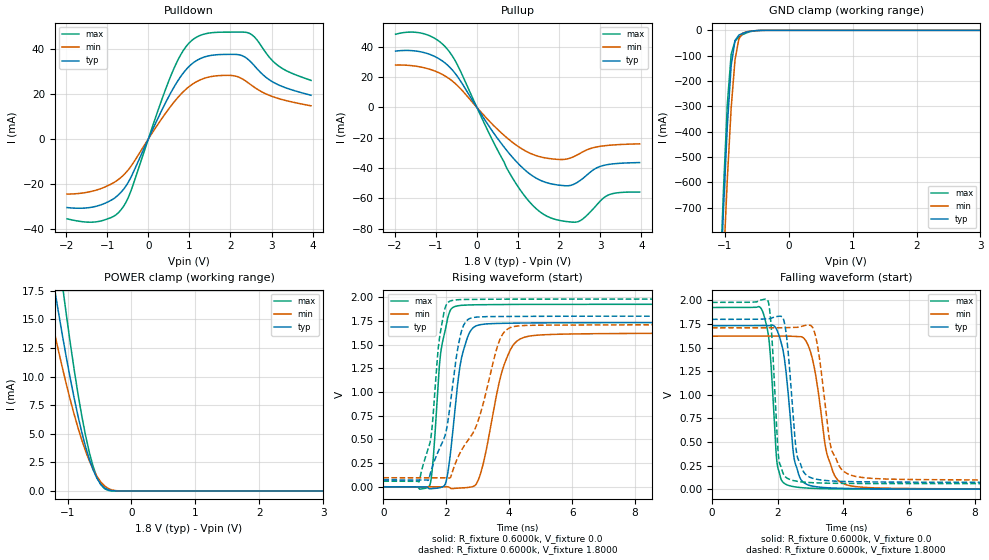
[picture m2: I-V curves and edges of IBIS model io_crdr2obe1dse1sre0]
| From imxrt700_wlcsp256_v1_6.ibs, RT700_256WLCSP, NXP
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[Model] io_crdr2obe1dse1sre0
|   Model io_crdr2obe1dse1sre0
| This model was characterised for following simulation conditions:
| External (pad) voltage:
|   - Typ: 1.8V,   - Min: 1.71V,   - Max: 1.98V
| Library cells for typ/min/max conditions are connected as defined below:
|  PAD_IO - External Pad
|  ipp_do - Core Input
|  ipp_obe - Output Buffer Enable
|  ASRCN3V3[3] - NC
|  ASRCN3V3[4] - NC
|  ASRCP3V3[4] - NC
|  REFAPBIAS3V3 - gnde
|  REFBAMPL3V3 - vdd1v8
|  REFCAMPH3V3 - vdd1v8
|  REFDNBIAS3V3 - vdd1v8
|  REFH3V3 - REFH3V3
|  REFL3V3 - REFL3V3
|  gnde - gnde
|  ipp_dse - vdd
|  ipp_ina235_3v - NC
|  ipp_ina40_3v - NC
|  ipp_ina_mux - NC
|  ipp_ind - NC
|  ipp_ind_1p8v - NC
|  ipp_ind_3v - NC
|  ipp_sre - gnde
|  vdd - vdd
|  vdd1v8 - vdd1v8
|  vdda - vdde3v3
|  vdde3v3 - vdde3v3
| All other pins connected to ground
Model_type I/O
Polarity   Non-Inverting
Enable   Active-High
Vinl =   0.5400V
Vinh =   1.2600V
Vmeas =  0.9000V
Cref =   15.0000pF
Rref =   0.6000k
Vref =   0.0V
C_comp   3.9792pF   3.7942pF   4.1043pF
|C_comp_pullup   0.4868pF   0.5823pF   0.4754pF
|C_comp_pulldown   2.0823pF   2.1675pF   1.8519pF
[Model Spec]
| variable   typ   min   max
Vinh   1.2600V   NA   NA
Vinl   0.5400V   NA   NA
Vref   0.0V   0.0V   0.0V
Cref   15.0000pF   15.0000pF   15.0000pF
Rref   0.6000k   0.6000k   0.6000k
[Receiver Thresholds]
Vcross_high  =   0.0V
Vcross_low  =   0.0V
Vdiff_ac  =   0.0V
Vdiff_dc  =   0.0V
Tdiffslew_ac  =   0.0S
[Temperature Range]   25.0000   0.1250k   -40.0000
[Voltage Range]   1.8000V   1.7100V   1.9800V
[Pullup Reference]   1.8000V   1.7100V   1.9800V
[Pulldown Reference]   0.0V   0.0V   0.0V
[POWER Clamp Reference]   1.8000V   1.7100V   1.9800V
[GND Clamp Reference]   0.0V   0.0V   0.0V
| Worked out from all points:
|   slope of the pulldown table from 0 to 0.27 V, typ, clamps not added: 25.6 ohm
|   slope of the pullup table from 0 to 0.27 V, typ, clamps not added: 23.8 ohm
|   GND clamp passes 1 mA (typ) near -0.50 V on its own axis
|   POWER clamp passes 1 mA (typ) near -0.53 V on its own axis
|   rising waveform, R_fixture 0.6000k, V_fixture 0.0: 20-80 % time 373ps typ, 622ps min, 283ps max; typ from 0 V to 1.73 V
|   rising waveform, R_fixture 0.6000k, V_fixture 1.8000: 20-80 % time 558ps typ, 1ns min, 331ps max; typ from 0.072 V to 1.8 V
|   falling waveform, R_fixture 0.6000k, V_fixture 0.0: 20-80 % time 288ps typ, 434ps min, 205ps max; typ from 1.73 V to 0 V
|   falling waveform, R_fixture 0.6000k, V_fixture 1.8000: 20-80 % time 243ps typ, 371ps min, 176ps max; typ from 1.8 V to 0.072 V
[Pulldown]
|Voltage   I(typ)   I(min)   I(max)
-1.98V    -30.4mA    -24.44mA   -35.4mA
-1.2V     -29.48mA   -22.28mA   -36.54mA
-840mV    -26.45mA   -19.34mA   -34.25mA
-600mV    -22.26mA   -15.94mA   -29.79mA
-420mV    -16.87mA   -12.03mA   -22.87mA
600mV     22.22mA    15.79mA    30.28mA
900mV     30.36mA    21.79mA    40.52mA
1.14V     34.38mA    25.06mA    44.79mA
1.98V     37.51mA    28.2mA     47.38mA
2.46V     34.79mA    24.52mA    46.85mA
3.12V     24.4mA     18.2mA     33.06mA
3.96V     19.37mA    14.7mA     25.97mA
[Pullup]
|Voltage   I(typ)   I(min)   I(max)
-1.98V    37.17mA    27.99mA    48.3mA
-1.26V    36mA       26.04mA    48.37mA
-720mV    28.06mA    19.81mA    38.46mA
-480mV    20.65mA    14.61mA    28.37mA
780mV     -30.13mA   -21.13mA   -42.58mA
1.2V      -41.94mA   -28.92mA   -59.68mA
1.62V     -48.87mA   -33.02mA   -70.4mA
2.16V     -51.62mA   -34.11mA   -75.13mA
2.46V     -49.1mA    -31.02mA   -75.32mA
2.88V     -40.32mA   -26.22mA   -65.36mA
3.18V     -37.66mA   -25.01mA   -57.94mA
3.96V     -36.33mA   -23.97mA   -55.79mA
[GND_clamp]
|Voltage   I(typ)   I(min)   I(max)
-1.98V    -7.543A    -7.6A      -7.897A
-1.08V    -1.077A    -1.286A    -1.025A
-1.02V    -705.3mA   -921.3mA   -628.8mA
-960mV    -377.1mA   -587.4mA   -291.7mA
-900mV    -139.2mA   -307mA     -94.38mA
-840mV    -40.12mA   -117mA     -42.82mA
-780mV    -18.81mA   -33.95mA   -26.13mA
-720mV    -11.86mA   -11.44mA   -16.78mA
-660mV    -7.061mA   -5.737mA   -9.992mA
-540mV    -1.684mA   -1.901mA   -2.15mA
-420mV    -207.1uA   -403.7uA   -160.6uA
3.96V     0A         0A         0A
[POWER_clamp]
|Voltage   I(typ)   I(min)   I(max)
-1.98V    46.79mA    35.94mA    61.38mA
-1.32V    21.77mA    16.85mA    28.91mA
-1.2V     17.57mA    13.71mA    23.33mA
-1.14V    15.55mA    12.2mA     20.62mA
-1.08V    13.59mA    10.75mA    17.99mA
-1.02V    11.7mA     9.353mA    15.46mA
-900mV    8.209mA    6.76mA     10.73mA
-720mV    3.898mA    3.511mA    4.887mA
-540mV    1.103mA    1.267mA    1.195mA
-420mV    244.5uA    429.3uA    190.6uA
-180mV    280.9nA    5.273uA    26.8nA
3.96V     0A         0A         0A
[Ramp]
| variable   typ   min   max
dV/dt_r  1.0396/0.3731n   0.9730/0.6216n   1.1554/0.2833n
dV/dt_f  1.0366/0.2435n   0.9689/0.3706n   1.1528/0.1761n
R_load = 0.6000k
[Rising Waveform]
R_fixture= 0.6000k
V_fixture= 0.0
V_fixture_min= 0.0
V_fixture_max= 0.0
|time   V(typ)   V(min)   V(max)
0s        47.1nV     1.315uV    17.96nV
1.471ns   -22.21mV   -562.7uV   13.41mV
1.567ns   -18.88mV   -613.1uV   224.8mV
1.859ns   -3.186mV   -474.1uV   1.492V
2.072ns   195.4mV    -2.356mV   1.812V
2.466ns   1.328V     -13.46mV   1.913V
3.042ns   1.707V     90.46mV    1.92V
4.045ns   1.726V     1.449V     1.923V
4.903ns   1.729V     1.599V     1.924V
60ns      1.733V     1.622V     1.926V
[Rising Waveform]
R_fixture= 0.6000k
V_fixture= 1.8000
V_fixture_min= 1.7100
V_fixture_max= 1.9800
|time   V(typ)   V(min)   V(max)
0s        72.29mV    95.11mV    58.66mV
1.137ns   71.88mV    95.04mV    54.32mV
1.517ns   168.9mV    94.58mV    531.9mV
1.749ns   375.8mV    94.76mV    1.474V
1.904ns   490.7mV    94.93mV    1.805V
2.304ns   1.329V     259.7mV    1.972V
2.689ns   1.764V     489.8mV    1.976V
3.697ns   1.796V     1.548V     1.979V
4.338ns   1.797V     1.698V     1.979V
60ns      1.8V       1.71V      1.98V
[Falling Waveform]
R_fixture= 0.6000k
V_fixture= 0.0
V_fixture_min= 0.0
V_fixture_max= 0.0
|time   V(typ)   V(min)   V(max)
0s        1.733V     1.622V     1.926V
1.53ns    1.734V     1.622V     1.894V
1.754ns   1.733V     1.621V     1.519V
1.96ns    1.7V       1.622V     353.4mV
2.504ns   320.2mV    1.62V      25.55mV
2.704ns   104.1mV    1.616V     16.53mV
3.049ns   33.01mV    1.394V     8.929mV
3.683ns   11.94mV    184.8mV    3.453mV
4.534ns   5.204mV    21.6mV     1.214mV
60ns      2.73uV     5.893uV    303.8nV
[Falling Waveform]
R_fixture= 0.6000k
V_fixture= 1.8000
V_fixture_min= 1.7100
V_fixture_max= 1.9800
|time   V(typ)   V(min)   V(max)
0s        1.8V       1.71V      1.98V
1.702ns   1.804V     1.71V      1.998V
2.021ns   1.833V     1.71V      363.6mV
2.156ns   1.818V     1.711V     175.9mV
2.555ns   436.8mV    1.715V     85.65mV
2.795ns   180.5mV    1.733V     74.59mV
3.166ns   106mV      1.606V     66.81mV
3.66ns    86.8mV     400.1mV    62.47mV
4.77ns    76.89mV    116.8mV    59.62mV
60ns      72.29mV    95.11mV    58.66mV
